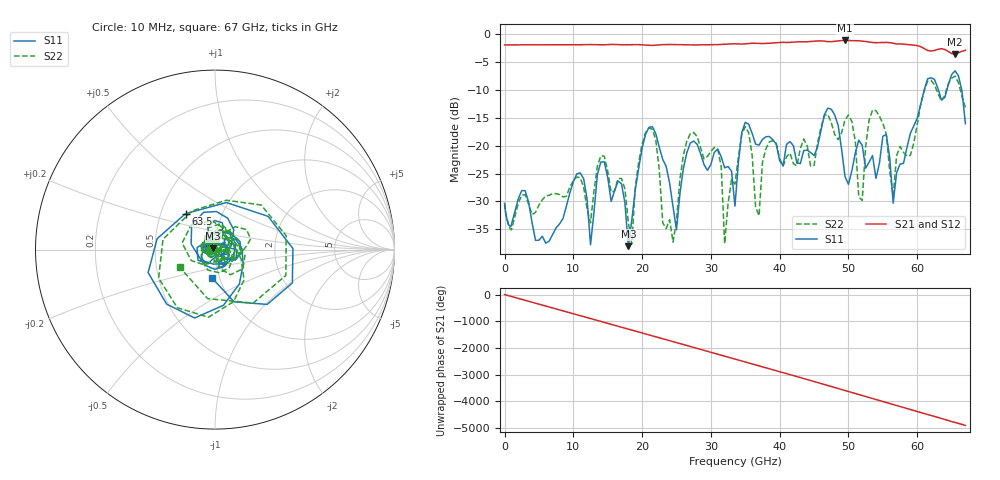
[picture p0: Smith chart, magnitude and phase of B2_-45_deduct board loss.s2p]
!Keysight Technologies,N5247B,MY61255065,A.16.20.04
!Date: Sunday, September 03, 2023 21:56:28
!Correction: S11(C  2-Port  )
!S21(C  2-Port  )
!S12(C  2-Port  )
!S22(C  2-Port  )
!S2P File: Measurements: S11, S21, S12, S22:
!Deduct Board Loss
# Hz S  dB  R 50
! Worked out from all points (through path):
!   142 points, 10 MHz to 67 GHz, reference 50 ohm
!   highest |S21| = -1.13 dB at 49.5 GHz (marker M1); lowest = -3.6 dB at 65.5 GHz (marker M2)
!   lowest |S11| = -38.0 dB at 18 GHz (marker M3), VSWR 1.03, Z = 48.9 + j0.632 ohm
!   |S11| at or under -10 dB: start of sweep to 61.02 GHz; 63.08 GHz to 64.31 GHz (1.23 GHz wide, 1.93 % of centre); 66.47 GHz to end of sweep
!   |S22| runs from -37.6 to -7.5 dB; largest |S21 - S12| = 0.0024
!   S11 on the Smith chart (normalised r, x): 10 MHz: 0.94, -0.01; 63.5 GHz: 0.67, +0.29; 67 GHz: 0.92, -0.30
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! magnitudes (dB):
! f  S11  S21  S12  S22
! 10 MHz  -30.3  -1.9  -1.9  -30.3
! 11.5 GHz  -25.9  -1.9  -1.9  -27.4
! 12.5 GHz  -37.8  -1.9  -1.9  -33.8
! 18 GHz  -38.0  -1.9  -1.9  -33.7
! 20.5 GHz  -18.0  -2.0  -2.0  -17.7
! 22.5 GHz  -20.3  -1.9  -1.9  -24.4
! 25 GHz  -35.1  -1.9  -1.9  -33.4
! 27 GHz  -19.5  -1.9  -1.9  -17.9
! 31 GHz  -20.6  -1.9  -1.9  -20.7
! 32 GHz  -23.9  -1.8  -1.8  -37.5
! 34 GHz  -23.0  -1.8  -1.8  -22.0
! 37 GHz  -19.9  -1.7  -1.7  -32.6
! 38.5 GHz  -18.4  -1.6  -1.6  -19.3
! 45 GHz  -21.8  -1.3  -1.3  -23.6
! 47.5 GHz  -13.5  -1.3  -1.3  -15.9
! 49.5 GHz  -25.6  -1.1  -1.1  -15.4
! 51.5 GHz  -19.0  -1.2  -1.2  -29.2
! 53.5 GHz  -21.8  -1.5  -1.5  -13.6
! 56 GHz  -22.2  -1.5  -1.5  -24.5
! 63.5 GHz  -11.7  -2.6  -2.6  -12.0
! 65.5 GHz  -6.6  -3.6  -3.6  -7.5
! 67 GHz  -16.0  -2.9  -2.9  -13.1
